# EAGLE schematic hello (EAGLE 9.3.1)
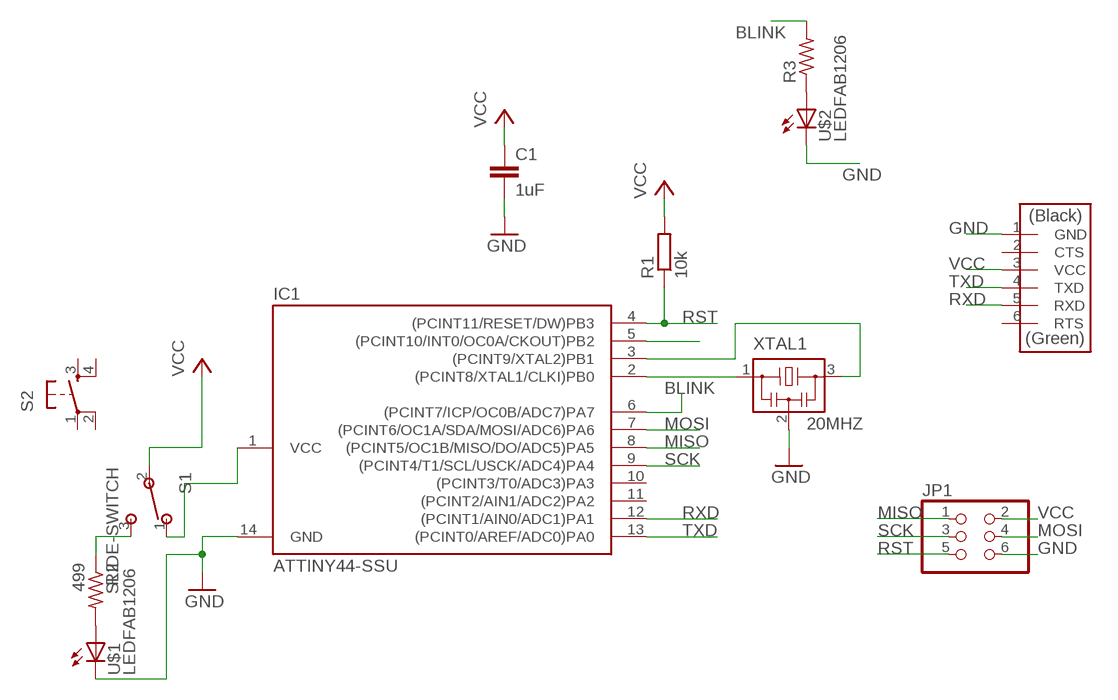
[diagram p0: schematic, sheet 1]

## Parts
C1  1uF  C-EUC1206  [C1206]
IC1  ATTINY44-SSU  [SOIC14]
J2  FTDI-SMD-HEADER  [1X06SMD]
JP1  PINHD-2X3-SMD  [2X03SMD]
R1  10k  R-EU_M1206  [M1206]
R2  499  RES-US1206FAB  [R1206FAB]
R3  RES-US1206FAB  [R1206FAB]
S1  SLIDE-SWITCH  [AYZ0102AGRLC]
S2  6MM_SWITCH6MM_SWITCH  [6MM_SWITCH]
U$1  LEDFAB1206  [LED1206FAB]
U$2  LEDFAB1206  [LED1206FAB]
XTAL1  20MHZ  RESONATOR  [EFOBM]

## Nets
BLINK: IC1.6((PCINT7/ICP/OC0B/ADC7)PA7) R3.2
GND: C1.2 IC1.14(GND) J2.1(GND) JP1.6 U$1.2(C) U$2.2(C) XTAL1.2
MISO: IC1.8((PCINT5/OC1B/MISO/DO/ADC5)PA5) JP1.1
MOSI: IC1.7((PCINT6/OC1A/SDA/MOSI/ADC6)PA6) JP1.4
N$1: IC1.1(VCC) S1.1
N$2: R2.1 S1.3
N$3: R2.2 U$1.1(A)
N$4: IC1.5((PCINT10/INT0/OC0A/CKOUT)PB2)
N$5: R3.1 U$2.1(A)
N$7: IC1.2((PCINT8/XTAL1/CLKI)PB0) XTAL1.1
N$8: IC1.3((PCINT9/XTAL2)PB1) XTAL1.3
RST: IC1.4((PCINT11/RESET/DW)PB3) JP1.5 R1.1
RXD: IC1.12((PCINT1/AIN0/ADC1)PA1) J2.5(RXD)
SCK: IC1.9((PCINT4/T1/SCL/USCK/ADC4)PA4) JP1.3
TXD: IC1.13((PCINT0/AREF/ADC0)PA0) J2.4(TXD)
VCC: C1.1 J2.3(VCC) JP1.2 R1.2 S1.2
Unconnected: IC1.10((PCINT3/T0/ADC3)PA3) IC1.11((PCINT2/AIN1/ADC2)PA2) J2.2(CTS) J2.6(RTS) S2.1(P) S2.2(P1) S2.3(S) S2.4(S1)

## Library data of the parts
C1 = rcl:C-EU: CAPACITOR, European symbol
IC1 = fab:ATTINY44
J2 = fab:FTDI-SMD-HEADER
JP1 = fab:PINHD-2X3-SMD: PIN HEADER
R1 = rcl:R-EU_: RESISTOR, European symbol
R2 R3 = fab:RES-US: Resistor (US Symbol)
S1 = fab:SLIDE-SWITCH: SMD slide-switch AYZ0102AGRLC as found in the fablab inventory. Includes the mounting holes. Made by Zaerc.
S2 = fab:6MM_SWITCH: OMRON SWITCH
U$1 U$2 = fab:LED: LED
XTAL1 = fab:RESONATOR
